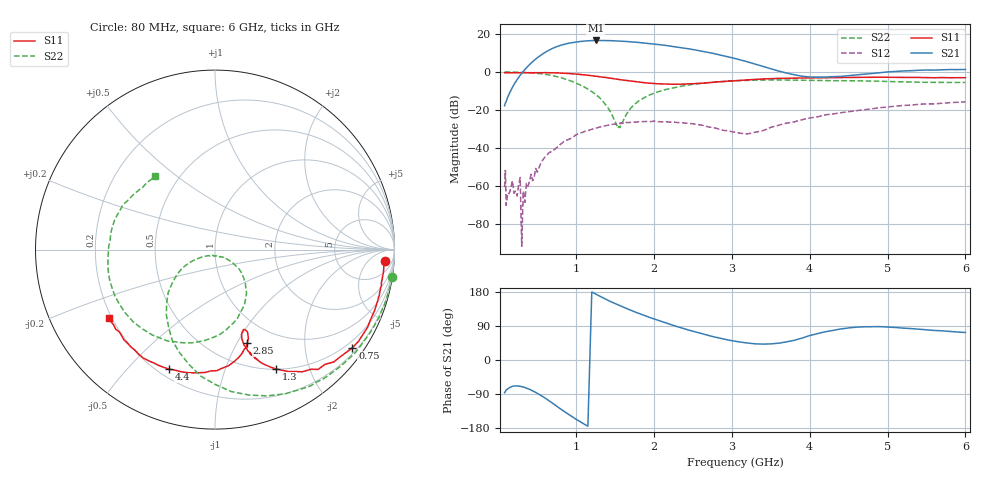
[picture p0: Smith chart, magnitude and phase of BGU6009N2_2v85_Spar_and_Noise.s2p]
! BGU6009N2, Vcc=2.85V, Icc= 5.7250 mA
# MHz S MA R 50
!  Freq-MHz  S11-mag  S11-arg  S21-mag  S21-arg  S12-mag  S12-arg  S22-mag  S22-arg
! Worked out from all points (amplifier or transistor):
!   130 points, 80 MHz to 6 GHz, reference 50 ohm
!   highest |S21| = 16.5 dB at 1.25 GHz (marker M1)
!   |S21| within 3 dB of that: 766.6 MHz to 2.217 GHz (1.451 GHz wide, 97.2 % of centre)
!   unconditionally stable (mu >= 1): start of sweep to 83.48 MHz; 97.47 MHz to end of sweep
!   at 480 MHz: K = 1.87, MAG = 23.3 dB, |S12| = -50.7 dB
!   at 1.615 GHz: K = 1.19, MAG = 18.8 dB, |S12| = -26.8 dB
!   at 6 GHz: K = 1.42, MAG = 4.7 dB, |S12| = -15.7 dB
!   lowest NFmin = 0.82 dB at 1.61 GHz
!   S11 on the Smith chart (normalised r, x): 80 MHz: 15, -18; 750 MHz: 0.32, -3.09; 1.3 GHz: 0.50, -1.51; 2.85 GHz: 0.74, -1.10; 4.4 GHz: 0.24, -0.66; 6 GHz: 0.19, -0.28
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80  0.9471 -3.7  0.1293 -86.2  0.0009403 -13.4  0.9968 -8.9
90  0.9471 -4.1  0.154 -83.2  0.002605 170.3  1 -10.0
100  0.9472 -4.6  0.1666 -79.3  0.0003162 -165.8  0.9986 -10.8
280  0.9492 -12.2  0.8168 -69.3  0.001692 -177.3  0.9749 -31.3
300  0.9463 -13.0  0.9186 -70.2  2.673e-05 -12.3  0.9723 -33.6
320  0.9487 -13.8  1.035 -71.3  0.0007457 -97.7  0.9705 -36.0
480  0.9515 -21.0  2.168 -85.6  0.002927 168.9  0.9276 -54.9
750  0.9408 -35.5  4.603 -122.1  0.01033 168.4  0.7512 -89.9
900  0.911 -43.4  5.64 -143.2  0.01682 161.0  0.6071 -109.0
1100  0.8373 -54.4  6.414 -168.9  0.02702 139.5  0.405 -131.8
1250  0.7716 -60.7  6.678 174.0  0.03322 128.9  0.2556 -146.5
1300  0.7466 -63.0  6.664 168.6  0.03556 123.5  0.2118 -150.4
1535  0.6384 -69.6  6.475 145.8  0.04426 106.4  0.03368 -110.8
1700  0.5734 -72.4  6.16 131.3  0.04748 95.7  0.1117 -36.4
2100  0.4833 -71.8  5.087 101.2  0.04898 73.5  0.3198 -57.7
2450  0.4874 -68.8  4.013 78.7  0.04411 61.9  0.4536 -82.5
2850  0.5512 -71.0  2.783 57.2  0.03083 58.7  0.5529 -110.6
3100  0.5976 -75.4  2.089 47.6  0.0247 74.0  0.5905 -126.4
4100  0.7029 -102.9  0.7315 69.8  0.06629 112.2  0.5953 -177.9
4400  0.7136 -110.9  0.7594 82.0  0.08473 108.4  0.588 171.1
5100  0.7161 -128.5  1.026 85.8  0.1259 95.7  0.5533 148.5
6000  0.7042 -147.3  1.159 72.6  0.1638 80.1  0.5285 129.6
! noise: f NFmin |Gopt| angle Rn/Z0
1000  0.83  0.3316  40.9  0.174
1250  0.8887  0.3421  47.79  0.1673
1505  0.8702  0.3326  52.6  0.1659
1535  0.8409  0.3379  52.73  0.1795
1560  0.9111  0.3387  54  0.1653
1590  0.8712  0.3295  54.09  0.1679
1620  0.8682  0.3338  55.69  0.1618
1645  0.8563  0.3295  56.47  0.1648
1900  0.865  0.3377  61.39  0.1767
2200  0.9714  0.3228  67.79  0.1726
